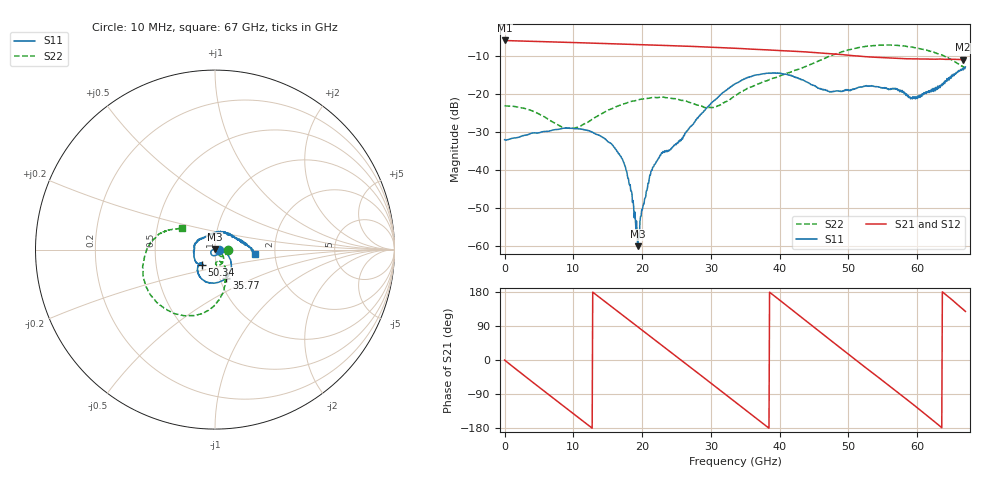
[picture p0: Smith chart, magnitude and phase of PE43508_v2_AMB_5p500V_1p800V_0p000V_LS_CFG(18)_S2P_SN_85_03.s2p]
!Keysight Technologies,N5227A,US51270237,A.10.43.00
!Date: Wednesday, August 22, 2018 17:08:24
!Correction: S11(Full 2 Port(1,3))
!S31(Full 2 Port(1,3))
!S13(Full 2 Port(1,3))
!S33(Full 2 Port(1,3))
!S2P File: Measurements: S11, S31, S13, S33:
# Hz S  dB  R 50
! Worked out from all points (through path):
!   801 points, 10 MHz to 67 GHz, reference 50 ohm
!   highest |S21| = -5.95 dB at 10 MHz (marker M1); lowest = -11.0 dB at 66.67 GHz (marker M2)
!   group delay of S21, straight-line fit = 39.2 ps
!   lowest |S11| = -60.2 dB at 19.35 GHz (marker M3), VSWR 1.00, Z = 50 + j0.0919 ohm
!   |S11| at or under -10 dB: start of sweep to end of sweep
!   |S22| runs from -29.1 to -7.1 dB; largest |S21 - S12| = 0.0032
!   S11 on the Smith chart (normalised r, x): 10 MHz: 1.05, -0.00; 35.77 GHz: 1.08, -0.34; 50.34 GHz: 0.85, -0.15; 67 GHz: 1.58, -0.08
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1e7  -32.11 -1.2  -5.95 -0.2  -5.95 -0.2  -23.13 -0.8
5.70415e9  -29.95 -74.0  -6.27 -81.4  -6.26 -81.3  -25.99 -49.6
8.300012e9  -29.17 -100.3  -6.41 -117.8  -6.40 -117.8  -28.71 -52.5
1.123082e10  -29.34 -124.3  -6.57 -158.8  -6.57 -158.8  -28.28 -38.4
1.399416e10  -31.12 -147.7  -6.73 162.7  -6.72 162.7  -25.35 -36.9
1.700871e10  -36.95 -174.0  -6.91 120.7  -6.90 120.7  -22.87 -48.1
1.818104e10  -44.07 177.4  -6.97 104.3  -6.96 104.4  -22.10 -53.3
1.935336e10  -60.16 110.4  -7.04 88.0  -7.03 88.1  -21.61 -59.3
2.119559e10  -41.49 -22.7  -7.15 62.3  -7.14 62.4  -21.09 -68.5
2.236791e10  -37.00 -26.9  -7.22 46.0  -7.22 46.0  -20.96 -74.1
2.714095e10  -28.46 -15.0  -7.52 -20.8  -7.51 -20.7  -22.41 -87.1
3.040671e10  -21.93 -23.0  -7.76 -66.7  -7.76 -66.6  -23.58 -72.5
3.3505e10  -17.43 -48.1  -8.01 -110.4  -8.01 -110.3  -20.56 -60.5
3.576591e10  -15.50 -67.9  -8.23 -142.2  -8.22 -142.1  -18.25 -61.1
3.978531e10  -14.60 -105.0  -8.59 161.1  -8.58 161.2  -15.52 -70.4
4.472582e10  -17.65 -136.1  -9.08 90.5  -9.06 90.6  -12.10 -80.2
5.033624e10  -18.92 -131.5  -9.90 10.3  -9.90 10.2  -8.27 -107.6
5.586291e10  -18.93 178.1  -10.57 -67.2  -10.59 -67.5  -7.14 -145.1
6.004979e10  -20.61 99.2  -10.81 -126.6  -10.85 -126.8  -8.03 -173.2
6.339929e10  -17.75 35.1  -10.85 -176.2  -10.92 -176.3  -9.70 165.6
6.666505e10  -13.71 -2.8  -11.03 133.5  -11.08 134.0  -12.86 148.9
6.7e10  -12.95 -5.9  -11.02 128.3  -11.07 128.6  -13.18 146.7
